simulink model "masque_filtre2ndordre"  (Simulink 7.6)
settings: Solver=ode45  StartTime=0.0  StopTime=10.0  RelTol=1e-3
libraries: powerlib_extras x1

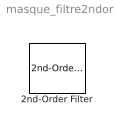
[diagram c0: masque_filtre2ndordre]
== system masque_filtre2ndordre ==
  2nd-Order Filter : powerlib_extras/Control  Blocks/2nd-Order Filter  DialogController=POWERSYS.PowerSysDialog  SystemSampleTime=-1  FilterType=Lowpass  Fo=200  Zeta=0.707  Initialize=off  Vac_Init=[1 45 60]  Vdc_Init=-0.5  PlotResponse=off  param1=[1 500 1]
